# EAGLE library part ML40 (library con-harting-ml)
HARTING
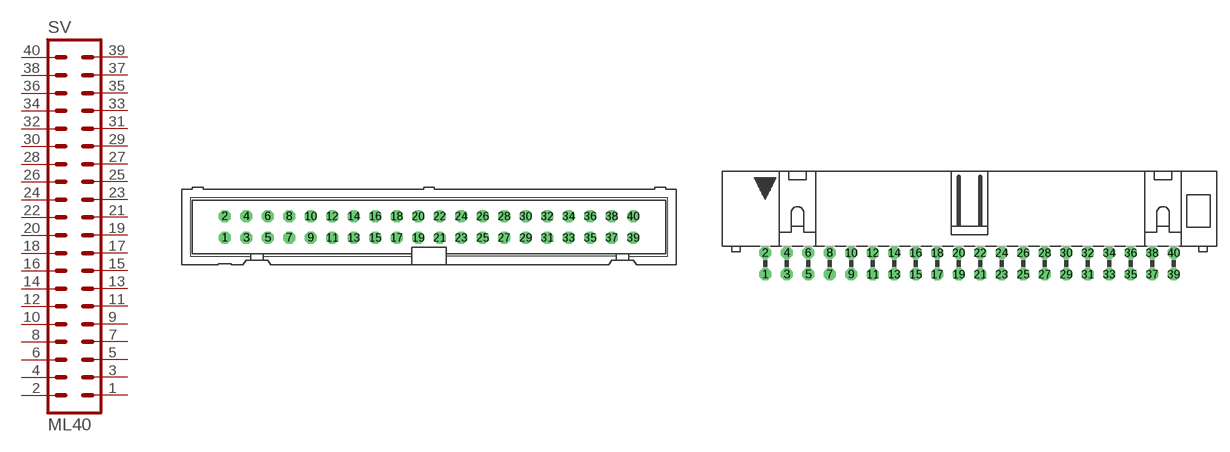
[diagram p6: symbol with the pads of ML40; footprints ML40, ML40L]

Designator prefix SV

## ML40 (OC_FARNELL: unknown; OC_NEWARK: unknown)  [ML40]
1  1  pas
2  2  pas
3  3  pas
4  4  pas
5  5  pas
6  6  pas
7  7  pas
8  8  pas
9  9  pas
10  10  pas
11  11  pas
12  12  pas
13  13  pas
14  14  pas
15  15  pas
16  16  pas
17  17  pas
18  18  pas
19  19  pas
20  20  pas
21  21  pas
22  22  pas
23  23  pas
24  24  pas
25  25  pas
26  26  pas
27  27  pas
28  28  pas
29  29  pas
30  30  pas
31  31  pas
32  32  pas
33  33  pas
34  34  pas
35  35  pas
36  36  pas
37  37  pas
38  38  pas
39  39  pas
40  40  pas

## ML40L (OC_FARNELL: unknown; OC_NEWARK: unknown)  [ML40L]
Pads as for ML40

## ML403M (OC_FARNELL: unknown; OC_NEWARK: unknown)  [3M_40]
Pads as for ML40

## ML403ML (OC_FARNELL: unknown; OC_NEWARK: unknown)  [3M_40L]
Pads as for ML40

## Footprint ML40 (pad centres in mm)
HARTING
drill 0.914 octagon: 1 -24.13,-1.27; 2 -24.13,1.27; 3 -21.59,-1.27; 4 -21.59,1.27; 5 -19.05,-1.27; 6 -19.05,1.27; 7 -16.51,-1.27; 8 -16.51,1.27; 9 -13.97,-1.27; 10 -13.97,1.27; 11 -11.43,-1.27; 12 -11.43,1.27; 13 -8.89,-1.27; 14 -8.89,1.27; 15 -6.35,-1.27; 16 -6.35,1.27; 17 -3.81,-1.27; 18 -3.81,1.27; 19 -1.27,-1.27; 20 -1.27,1.27; 21 1.27,-1.27; 22 1.27,1.27; 23 3.81,-1.27; 24 3.81,1.27; 25 6.35,-1.27; 26 6.35,1.27; 27 8.89,-1.27; 28 8.89,1.27; 29 11.43,-1.27; 30 11.43,1.27; 31 13.97,-1.27; 32 13.97,1.27; 33 16.51,-1.27; 34 16.51,1.27; 35 19.05,-1.27; 36 19.05,1.27; 37 21.59,-1.27; 38 21.59,1.27; 39 24.13,-1.27; 40 24.13,1.27

## Footprint ML40L (pad centres in mm)
HARTING
drill 0.914 octagon: 1 -24.13,-1.27; 2 -24.13,1.27; 3 -21.59,-1.27; 4 -21.59,1.27; 5 -19.05,-1.27; 6 -19.05,1.27; 7 -16.51,-1.27; 8 -16.51,1.27; 9 -13.97,-1.27; 10 -13.97,1.27; 11 -11.43,-1.27; 12 -11.43,1.27; 13 -8.89,-1.27; 14 -8.89,1.27; 15 -6.35,-1.27; 16 -6.35,1.27; 17 -3.81,-1.27; 18 -3.81,1.27; 19 -1.27,-1.27; 20 -1.27,1.27; 21 1.27,-1.27; 22 1.27,1.27; 23 3.81,-1.27; 24 3.81,1.27; 25 6.35,-1.27; 26 6.35,1.27; 27 8.89,-1.27; 28 8.89,1.27; 29 11.43,-1.27; 30 11.43,1.27; 31 13.97,-1.27; 32 13.97,1.27; 33 16.51,-1.27; 34 16.51,1.27; 35 19.05,-1.27; 36 19.05,1.27; 37 21.59,-1.27; 38 21.59,1.27; 39 24.13,-1.27; 40 24.13,1.27

## Footprint 3M_40 (pad centres in mm)
3M
drill 0.813 square: 1 -24.13,-1.27; 2 -24.13,1.27; 3 -21.59,-1.27; 4 -21.59,1.27; 5 -19.05,-1.27; 6 -19.05,1.27; 7 -16.51,-1.27; 8 -16.51,1.27; 9 -13.97,-1.27; 10 -13.97,1.27; 11 -11.43,-1.27; 12 -11.43,1.27; 13 -8.89,-1.27; 14 -8.89,1.27; 15 -6.35,-1.27; 16 -6.35,1.27; 17 -3.81,-1.27; 18 -3.81,1.27; 19 -1.27,-1.27; 20 -1.27,1.27; 21 1.27,-1.27; 22 1.27,1.27; 23 3.81,-1.27; 24 3.81,1.27; 25 6.35,-1.27; 26 6.35,1.27; 27 8.89,-1.27; 28 8.89,1.27; 29 11.43,-1.27; 30 11.43,1.27; 31 13.97,-1.27; 32 13.97,1.27; 33 16.51,-1.27; 34 16.51,1.27; 35 19.05,-1.27; 36 19.05,1.27; 37 21.59,-1.27; 38 21.59,1.27; 39 24.13,-1.27; 40 24.13,1.27

## Footprint 3M_40L (pad centres in mm)
3M
drill 0.813 square: 1 -24.13,-5.08; 2 -24.13,-2.54; 3 -21.59,-5.08; 4 -21.59,-2.54; 5 -19.05,-5.08; 6 -19.05,-2.54; 7 -16.51,-5.08; 8 -16.51,-2.54; 9 -13.97,-5.08; 10 -13.97,-2.54; 11 -11.43,-5.08; 12 -11.43,-2.54; 13 -8.89,-5.08; 14 -8.89,-2.54; 15 -6.35,-5.08; 16 -6.35,-2.54; 17 -3.81,-5.08; 18 -3.81,-2.54; 19 -1.27,-5.08; 20 -1.27,-2.54; 21 1.27,-5.08; 22 1.27,-2.54; 23 3.81,-5.08; 24 3.81,-2.54; 25 6.35,-5.08; 26 6.35,-2.54; 27 8.89,-5.08; 28 8.89,-2.54; 29 11.43,-5.08; 30 11.43,-2.54; 31 13.97,-5.08; 32 13.97,-2.54; 33 16.51,-5.08; 34 16.51,-2.54; 35 19.05,-5.08; 36 19.05,-2.54; 37 21.59,-5.08; 38 21.59,-2.54; 39 24.13,-5.08; 40 24.13,-2.54
hole 2.54 at -30.048,-3.277
hole 2.54 at 30.048,-3.277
